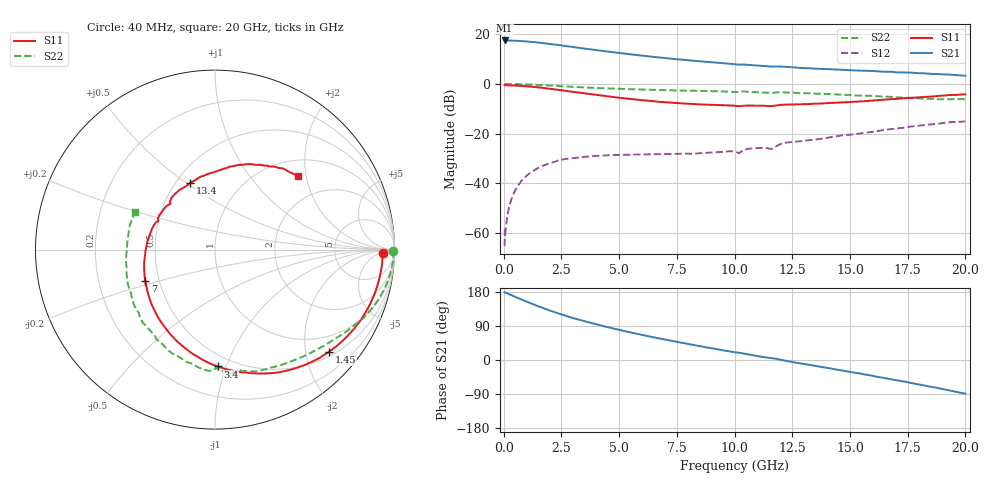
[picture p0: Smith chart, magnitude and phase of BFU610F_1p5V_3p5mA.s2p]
! Filename:  P:\Prog\Test\Noise\ATS_data\Testdata_Net\SplitFiles\BFU610_2W_A5_HighFreq_1.5V_3.5mA_D.s2p
! Date/Time: Wed 10/Aug/2011 16:54:08
! BFU610_2W_A5_HighFreq_Bias3_1.5V_1mA_10mA_R.s2p
! MDIF S-parameter v. bias file
! BFU610_2W_A5_HighFreq_1.5V_1mA_10mA
! Date/time Mon Aug 08 13:57:57 2011
! VAR V_out= 1.5001
! VAR I_out= 3.4950
! VAR V_in= 0.8900
! VAR I_in= 0.0277
! Device data file deembeded for feedlines and parallel
! Original file: \SplitFiles\BFU610_2W_A5_HighFreq_1.5V_3.5mA_R.s2p
! Feed-files: PR003V01_101208_Feed1.s2p, PR003V01_101208_Feed2.s2p
! Parallel-file: PR003V01_101208_Par.s2p
# MHz S MA R 50
!  Freq-MHz  S11-mag  S11-arg  S21-mag  S21-arg  S12-mag  S12-arg  S22-mag  S22-arg
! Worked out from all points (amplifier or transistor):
!   167 points, 40 MHz to 20 GHz, reference 50 ohm
!   highest |S21| = 17.4 dB at 40 MHz (marker M1)
!   |S21| within 3 dB of that: start of sweep to 3.286 GHz
!   unconditionally stable (mu >= 1): 5.409 GHz to 18.68 GHz
!   at 550 MHz: K = 0.04, MSG = 29.6 dB, |S12| = -42.0 dB
!   at 4.2 GHz: K = 0.75, MSG = 21.1 dB, |S12| = -28.9 dB
!   at 20 GHz: K = 0.90, MSG = 9.2 dB, |S12| = -15.1 dB
!   S11 on the Smith chart (normalised r, x): 40 MHz: 27, -8; 1.45 GHz: 0.59, -2.49; 3.4 GHz: 0.41, -0.94; 7 GHz: 0.42, -0.18; 13.4 GHz: 0.59, +0.52; 20 GHz: 1.35, +1.78
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40  0.9349 -1.2  7.443 178.9  0.0005437 85.9  0.9932 -0.3
50  0.9313 -1.3  7.416 178.9  0.001147 99.8  0.9934 -0.5
70  0.9354 -2.0  7.403 178.1  0.0009318 88.9  0.9944 -0.7
200  0.9335 -6.0  7.391 174.6  0.002804 89.5  0.994 -2.4
380  0.9283 -11.4  7.369 169.8  0.005471 86.3  0.9919 -4.6
950  0.8954 -28.1  7.142 155.1  0.01361 74.5  0.9749 -11.4
1450  0.8528 -42.0  6.796 143.0  0.01983 65.2  0.952 -16.9
1850  0.8129 -52.6  6.476 133.8  0.02399 58.7  0.9309 -21.0
2250  0.7702 -62.7  6.132 125.2  0.02741 53.9  0.9094 -25.0
2800  0.7085 -75.5  5.666 114.6  0.03133 45.0  0.8773 -29.4
3400  0.6513 -88.6  5.188 104.1  0.0336 39.8  0.8488 -34.1
4100  0.5902 -103.0  4.709 92.7  0.03579 34.5  0.8211 -39.0
4900  0.5316 -118.2  4.222 80.9  0.03705 30.3  0.7956 -44.4
5800  0.4783 -134.8  3.771 68.7  0.03792 27.3  0.7721 -50.4
6800  0.4333 -152.3  3.358 56.2  0.03847 26.0  0.7503 -56.9
7000  0.4264 -155.7  3.286 53.8  0.03864 26.0  0.7458 -58.2
8600  0.3834 177.8  2.818 35.5  0.04037 28.7  0.7207 -68.9
10200  0.3542 153.0  2.43 19.2  0.04045 33.5  0.6863 -78.4
12000  0.3772 130.1  2.224 0.5  0.06194 41.6  0.6763 -92.8
13400  0.3971 110.4  2.028 -14.5  0.07496 32.8  0.6367 -106.4
16800  0.4921 73.8  1.742 -51.0  0.1229 15.8  0.545 -146.4
20000  0.6158 41.6  1.454 -88.9  0.1756 -14.8  0.492 154.8
